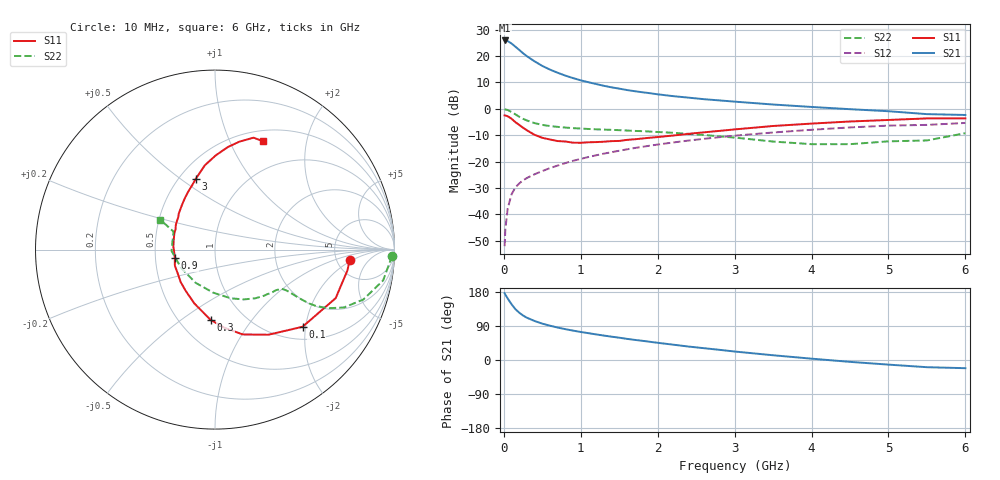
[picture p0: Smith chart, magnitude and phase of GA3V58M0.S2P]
! Infineon Technologies  Discrete & RF Semiconductors
! BF775
! Si NPN RF Bipolar Junction Transistor in SOT23
! VCE = 3.5 V  IC = 8 mA
! Common Emitter S-Parameters:  May  1996
# GHz  S  MA  R  50
!  f  S11  S21  S12  S22
! GHz  MAG  ANG  MAG  ANG  MAG  ANG  MAG  ANG
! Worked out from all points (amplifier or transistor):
!   36 points, 10 MHz to 6 GHz, reference 50 ohm
!   highest |S21| = 25.9 dB at 10 MHz (marker M1)
!   |S21| within 3 dB of that: start of sweep to 176 MHz
!   unconditionally stable (mu >= 1): 643.4 MHz to 3.26 GHz
!   at 250 MHz: K = 0.62, MSG = 24.1 dB, |S12| = -27.1 dB
!   at 1.4 GHz: K = 1.12, MAG = 10.2 dB, |S12| = -16.4 dB
!   at 6 GHz: K = 0.95, MSG = 1.5 dB, |S12| = -5.3 dB
!   S11 on the Smith chart (normalised r, x): 10 MHz: 6.60, -1.76; 100 MHz: 1.29, -1.92; 300 MHz: 0.70, -0.65; 900 MHz: 0.63, -0.06; 3 GHz: 0.60, +0.57; 6 GHz: 0.63, +1.34
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0.01  0.7525 -4.4  19.79 176.3  0.0025 85.8  0.9866 -2.0
0.02  0.747 -8.9  19.61 172.4  0.0053 82.1  0.9761 -4.2
0.05  0.7248 -21.9  19.25 162.3  0.0129 79.8  0.9524 -10.4
0.1  0.6502 -41.4  17.31 147.2  0.024 71.3  0.872 -18.6
0.15  0.5599 -57.9  15.07 134.2  0.0324 65.6  0.7871 -24.2
0.2  0.4973 -71.9  13.1 124.9  0.0386 62.3  0.7097 -27.4
0.25  0.4385 -83.2  11.31 117.4  0.0443 60.6  0.6472 -29.1
0.3  0.3926 -93.5  9.942 111.5  0.049 60.4  0.6027 -29.8
0.4  0.3218 -110.8  7.947 102.9  0.0577 60.3  0.5372 -30.0
0.5  0.2828 -125.0  6.512 95.9  0.0662 61.1  0.4965 -29.8
0.6  0.2629 -136.8  5.544 90.5  0.0754 61.5  0.4724 -29.7
0.7  0.2451 -148.8  4.833 85.6  0.0843 62.1  0.4557 -29.8
0.9  0.2286 -168.0  3.828 77.5  0.1037 62.5  0.4313 -30.5
1.1  0.2326 176.2  3.199 70.8  0.1224 62.4  0.4159 -32.5
1.3  0.2385 163.6  2.737 64.5  0.1417 61.6  0.4044 -34.6
1.6  0.2584 147.6  2.276 55.8  0.171 59.5  0.3887 -39.0
2.2  0.3123 125.7  1.743 40.5  0.2306 54.4  0.3521 -50.4
3  0.4079 105.3  1.371 22.4  0.3102 45.5  0.2855 -72.0
3.5  0.4737 96.8  1.209 12.5  0.3566 39.3  0.2402 -92.3
4.5  0.5762 82.8  0.986 -4.9  0.4448 26.2  0.2144 -151.1
5.5  0.6594 71.0  0.795 -19.0  0.4968 11.5  0.2521 156.5
6  0.6608 65.9  0.766 -21.6  0.5413 7.4  0.3462 151.4
